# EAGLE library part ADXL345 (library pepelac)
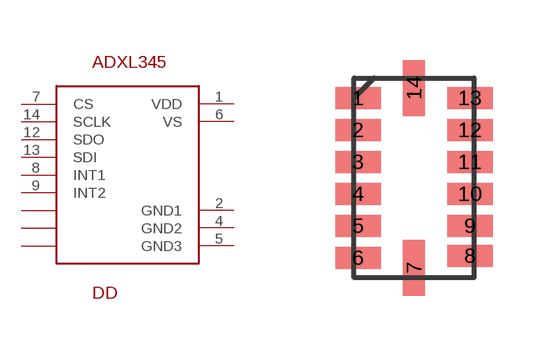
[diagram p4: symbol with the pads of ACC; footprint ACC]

Designator prefix DD

## ADXL345  [ACC]
1  VDD
2  GND1
3  P$1
4  GND2
5  GND3
6  VS
7  CS
8  INT1
9  INT2
10  P$2
11  P$3
12  SDO
13  SDI
14  SCLK

## Footprint ACC (pad centres in mm)
smd 1.145 x 0.55: 1 -1.4,2; 2 -1.4,1.2; 3 -1.4,0.4; 4 -1.4,-0.4; 5 -1.4,-1.2; 6 -1.4,-2; 8 1.4,-1.95; 9 1.4,-1.2; 10 1.4,-0.4; 11 1.4,0.4; 12 1.4,1.2; 13 1.4,2
smd 0.55 x 1.4: 7 0,-2.25; 14 0,2.25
